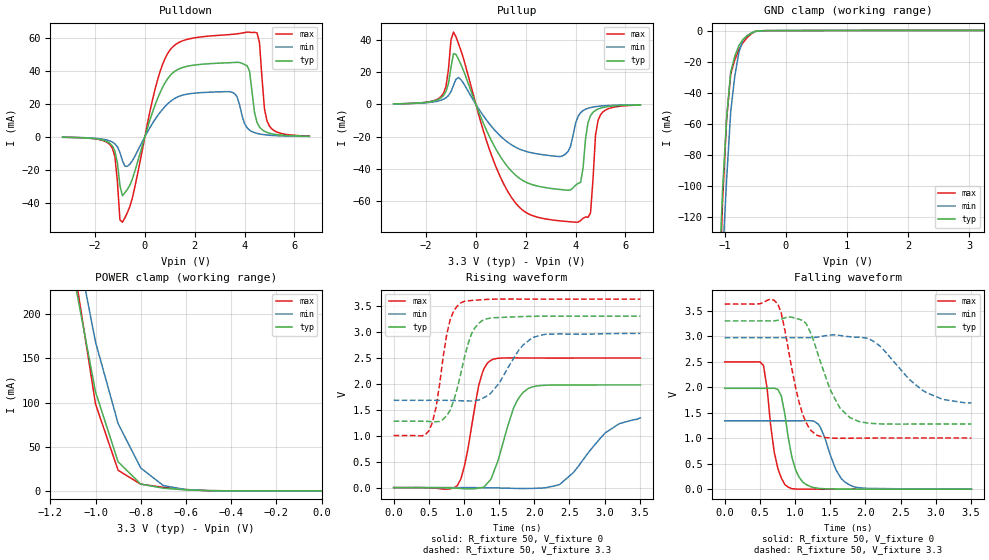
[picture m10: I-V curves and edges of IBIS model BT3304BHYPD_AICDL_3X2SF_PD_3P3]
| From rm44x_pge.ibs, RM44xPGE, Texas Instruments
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|   Model Cell BT3304BHYPD_AICDL_3X2SF_PD_3P3
|BT3304BHYPD_AICDL_3X2SF_PD_3P3
[Model]   BT3304BHYPD_AICDL_3X2SF_PD_3P3
Model_type   I/O
Polarity   Non-Inverting
Enable   Active-Low
Vinl =  1.15
Vinh =  1.55
Cref =  15.0001pF
Rref =  101.0000M
Vref =  0V
Vmeas =  1.65
C_comp   1.2p   1.2p   1.2p
[Model Spec]
Vinl   1.15   1.02   1.28
Vinh   1.55   1.45   1.65
[Temperature Range]   25   155   -40
[Voltage Range]   3.3   2.97   3.63
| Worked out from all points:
|   slope of the pulldown table from 0 to 0.495 V, typ, clamps not added: 22 ohm
|   slope of the pullup table from 0 to 0.495 V, typ, clamps not added: 26.9 ohm
|   GND clamp passes 1 mA (typ) near -0.53 V on its own axis
|   POWER clamp passes 1 mA (typ) near -0.58 V on its own axis
|   rising waveform, R_fixture 50, V_fixture 0: 20-80 % time 273ps typ, 493ps min, 197ps max; typ from 0 V to 1.98 V
|   rising waveform, R_fixture 50, V_fixture 3.3: 20-80 % time 235ps typ, 364ps min, 182ps max; typ from 1.28 V to 3.3 V
|   falling waveform, R_fixture 50, V_fixture 0: 20-80 % time 165ps typ, 226ps min, 140ps max; typ from 1.98 V to 0 V
|   falling waveform, R_fixture 50, V_fixture 3.3: 20-80 % time 335ps typ, 534ps min, 237ps max; typ from 3.3 V to 1.28 V
[POWER_clamp]
|   voltage   I(typ)   I(min)   I(max)
-3.3V     4.054A     4.63A      4.887A
-1.1V     248.3mA    301mA      262.8mA
-1.067V   203mA      256.9mA    208mA
-1.033V   157.6mA    212.7mA    153.2mA
-1V       112.2mA    168.6mA    98.42mA
-900mV    32.96mA    76.25mA    23.38mA
-800mV    7.8mA      25.98mA    7.643mA
-700mV    3.129mA    6.08mA     4.158mA
-600mV    1.184mA    1.572mA    1.593mA
-500mV    283.5uA    413uA      371.9uA
0V        96.5uA     44.21uA    168.6uA
[Pulldown]
|   voltage   I(typ)   I(min)   I(max)
-3.3V     -289uA     -253.9uA   -287.1uA
-1.4V     -4mA       -2.489mA   -4.76mA
-1.2V     -8.69mA    -4.261mA   -12.05mA
-1V       -29.49mA   -9.376mA   -50.19mA
-900mV    -35.6mA    -14.42mA   -51.6mA
1V        36.78mA    21.07mA    52.28mA
3.5V      44.86mA    26.91mA    61.93mA
4.1V      42.98mA    5.456mA    63.29mA
4.6V      5.887mA    1.718mA    56.92mA
4.8V      3.323mA    1.257mA    16.92mA
5V        2.171mA    957.9uA    6.458mA
6.6V      331.3uA    239.5uA    466.8uA
[Pullup]
|   voltage   I(typ)   I(min)   I(max)
-3.3V     325.3uA    297.6uA    301.6uA
-1.4V     4.042mA    2.556mA    4.795mA
-1.2V     7.932mA    4.062mA    11.13mA
-900mV    31.45mA    11.76mA    44.76mA
1.4V      -40.91mA   -24.77mA   -56.99mA
3.4V      -52.76mA   -32.29mA   -72.18mA
4V        -50.08mA   -11.8mA    -72.98mA
4.2V      -48.37mA   -5.201mA   -71.98mA
4.6V      -7.019mA   -1.989mA   -67.23mA
4.8V      -3.708mA   -1.414mA   -19.03mA
5V        -2.349mA   -1.055mA   -6.475mA
6.6V      -340.9uA   -258.1uA   -448.7uA
[GND_clamp]
|   voltage   I(typ)   I(min)   I(max)
-3.3V     -3.25A     -2.875A    -4.945A
-1.1V     -166.9mA   -205.1mA   -187mA
-1.033V   -102.8mA   -146.7mA   -110.1mA
-966.7mV  -55.97mA   -95.69mA   -57.03mA
-900mV    -26.57mA   -52.04mA   -27.82mA
-833.3mV  -16.53mA   -29.29mA   -18.83mA
-766.7mV  -9.588mA   -13.93mA   -12.15mA
-700mV    -5.749mA   -5.945mA   -7.796mA
-566.7mV  -1.617mA   -1.656mA   -2.13mA
-500mV    -447.1uA   -618.6uA   -527.1uA
-366.7mV  -51.38uA   -77.06uA   -66.68uA
3.233V    96.49uA    48.3uA     168.5uA
[Ramp]
| variable   typ   min   max
dV/dt_f   1.260622/0.3437926n  0.8111907/0.5624418n   1.637946/0.2453328n
dV/dt_r   1.201741/0.2766966n  0.8156721/0.5018929n   1.515603/0.1986888n
R_load = 50
[Rising Waveform]
R_fixture = 50
V_fixture = 0
V_fixture_min = 0
V_fixture_max = 0
|   time   V(typ)   V(min)   V(max)
0s        -5.652uV   -2.766uV   -3.329uV
904ps     -12.99mV   203.2uV    38.41mV
1.008ns   -23.65mV   251.5uV    426.8mV
1.208ns   -11.25mV   -1.183mV   1.957V
1.408ns   247.4mV    -4.992mV   2.468V
1.712ns   1.556V     -14.56mV   2.496V
1.908ns   1.903V     -16.09mV   2.494V
2.36ns    1.975V     58.71mV    2.493V
3.008ns   1.976V     1.052V     2.494V
3.508ns   1.976V     1.34V      2.494V
[Rising Waveform]
R_fixture = 50
V_fixture = 3.3
V_fixture_min = 2.97
V_fixture_max = 3.63
|   time   V(typ)   V(min)   V(max)
0s        1.278V     1.68V      1.003V
504ps     1.272V     1.68V      1.1V
604ps     1.268V     1.68V      1.555V
756ps     1.388V     1.679V     2.957V
804ps     1.488V     1.678V     3.233V
956ps     2.2V       1.671V     3.556V
1.108ns   2.964V     1.666V     3.602V
1.284ns   3.236V     1.731V     3.619V
1.972ns   3.296V     2.886V     3.628V
3.508ns   3.298V     2.968V     3.628V
[Falling Waveform]
R_fixture = 50
V_fixture = 0
V_fixture_min = 0
V_fixture_max = 0
|   time   V(typ)   V(min)   V(max)
0s        1.977V     1.34V      2.494V
552ps     1.976V     1.34V      2.421V
704ps     1.978V     1.34V      727.1mV
804ps     1.832V     1.34V      222.2mV
904ps     1.007V     1.34V      38.94mV
1.056ns   239mV      1.34V      267.2uV
1.26ns    33.7mV     1.337V     633.1uV
1.584ns   3.333mV    374.1mV    423.8uV
1.776ns   1.524mV    82.51mV    465.3uV
3.508ns   289.5uV    529.7uV    25.74uV
[Falling Waveform]
R_fixture = 50
V_fixture = 3.3
V_fixture_min = 2.97
V_fixture_max = 3.63
|   time   V(typ)   V(min)   V(max)
0s        3.298V     2.969V     3.628V
756ps     3.309V     2.969V     3.629V
804ps     3.331V     2.969V     3.449V
1.108ns   3.307V     2.969V     1.468V
1.308ns   2.723V     2.978V     1.057V
1.512ns   1.918V     3.022V     1.003V
1.776ns   1.406V     2.987V     998.9mV
2.164ns   1.283V     2.851V     1.002V
2.88ns    1.277V     1.886V     1.003V
3.508ns   1.278V     1.69V      1.003V
